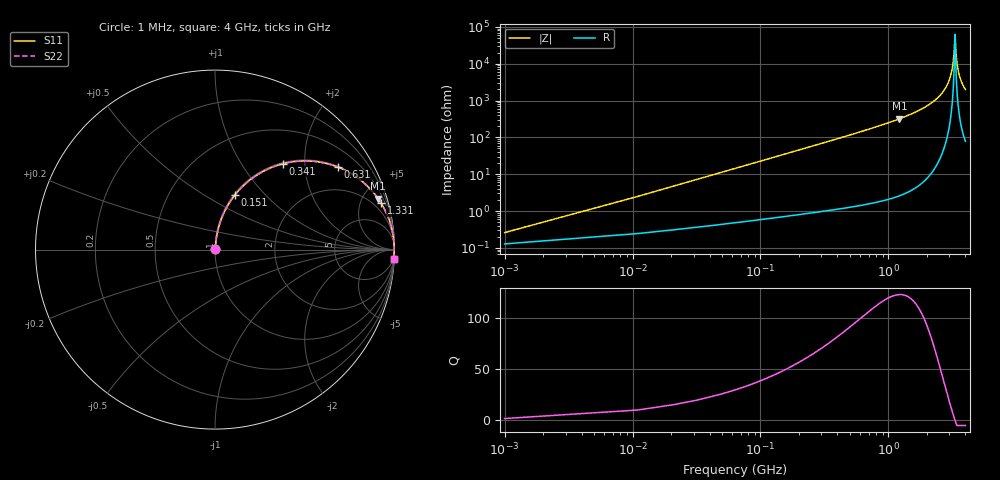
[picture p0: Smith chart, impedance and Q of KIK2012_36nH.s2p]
!version-2
!date-01.2022
!Series
# MHz S RI R 50
!Freq ReS11 ImS11 ReS21 ImS21 ReS12 ImS12 ReS22 ImS22
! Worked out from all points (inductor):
!   401 points, 1 MHz to 4 GHz, reference 50 ohm
!   read as one part in series: L = 36 nH near 21 MHz
!   highest Q = 123 at 1.221 GHz (marker M1), where L = 41.6 nH
!   self-resonance near 3.311 GHz
!   S11 on the Smith chart (normalised r, x): 1 MHz: 1.00, +0.00; 151 MHz: 1.01, +0.68; 341 MHz: 1.02, +1.56; 631 MHz: 1.03, +2.96; 1.331 GHz: 1.06, +7.18; 4 GHz: 3, -40
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1  0.00128 0.00226  0.9987 -0.00226  0.9987 -0.00226  0.00128 0.00226
31  0.00842 0.0693  0.9916 -0.0693  0.9916 -0.0693  0.00842 0.0693
41  0.0124 0.0912  0.9876 -0.0912  0.9876 -0.0912  0.0124 0.0912
81  0.0373 0.1755  0.9627 -0.1755  0.9627 -0.1755  0.0373 0.1755
151  0.1098 0.3026  0.8902 -0.3026  0.8902 -0.3026  0.1098 0.3026
341  0.3796 0.4787  0.6204 -0.4787  0.6204 -0.4787  0.3796 0.4787
631  0.6851 0.4596  0.3149 -0.4596  0.3149 -0.4596  0.6851 0.4596
671  0.7128 0.4477  0.2872 -0.4477  0.2872 -0.4477  0.7128 0.4477
1221  0.9089 0.2838  0.0911 -0.2838  0.0911 -0.2838  0.9089 0.2838
1331  0.9261 0.2575  0.0739 -0.2575  0.0739 -0.2575  0.9261 0.2575
1341  0.9275 0.2553  0.0725 -0.2553  0.0725 -0.2553  0.9275 0.2553
2001  0.9792 0.1375  0.0208 -0.1375  0.0208 -0.1375  0.9792 0.1375
2671  0.9952 0.0579  0.00479 -0.0579  0.00479 -0.0579  0.9952 0.0579
2921  0.9974 0.0339  0.00262 -0.0339  0.00262 -0.0339  0.9974 0.0339
3101  0.9982 0.018  0.00184 -0.018  0.00184 -0.018  0.9982 0.018
3221  0.9984 0.00792  0.00162 -0.00792  0.00162 -0.00792  0.9984 0.00792
3311  0.9984 0.0006  0.00159 -0.0006  0.00159 -0.0006  0.9984 0.0006
3341  0.9984 -0.0018  0.00161 0.0018  0.00161 0.0018  0.9984 -0.0018
3411  0.9983 -0.0073  0.00169 0.0073  0.00169 0.0073  0.9983 -0.0073
3531  0.998 -0.0165  0.00196 0.0165  0.00196 0.0165  0.998 -0.0165
3721  0.9973 -0.0304  0.00272 0.0304  0.00272 0.0304  0.9973 -0.0304
4000  0.9956 -0.0497  0.00444 0.0497  0.00444 0.0497  0.9956 -0.0497
